| TEXAS INSTRUMENTS INCORPORATED
| Standard Linear and Logic Group
| IBIS Model of SN74AHC138
| 3-LINE TO 8-LINE DECODERS/DEMULTIPLEXERS
| This file contains package information for the following:
|  QFN 16-pin (RGY) package as [Component] AHC138_RGY
|  PDIP 16-pin (N) package as [Component] AHC138_N
|  SOIC 16-pin (D) package as [Component] AHC138_D
|  SOP 16-pin (NS) package as [Component] AHC138_NS
|  SSOP 16-pin (DB) package as [Component] AHC138_DB
|  TSSOP 16-pin (PW) package as [Component] AHC138_PW
|  TVSOP 16-pin (DGV) package as [Component] AHC138_DGV
| This device can be powered at the following Vccs:
|  5 volt Vcc
|  3.3 volt Vcc
| This file provides unique models under the [Model Selector] for each Vcc.
| For operation at a specific Vcc, select the appropriate model after each
| [Model Selector] keyword.
[IBIS Ver]   3.2
[Comment char]  |_char
[File Name]   sn74ahc138.ibs
[File Rev]   1.1 | a_die
[Date]   April 5, 2006
[Source]   Data created from TI-SPICE simulations at TI-SLL.
[Notes]   The following is an IBIS list for the SN74AHC138.
   Please contact sllibis@ti.com with questions and
   comments concerning SLL IBIS models.
   - FILE REV HISTORY
   - 1.1 Release IBIS file on 04/10/06
   - C_comp values are taken at a different test condition
   than the data sheet.
   - Power clamp data deleted as there is no power-clamp diode.
[Disclaimer] Property of Texas Instruments Incorporated.  Unauthorized
   reproduction and/or distribution is strictly prohibited.
   This product is protected under copyright law.
   Created  2006, (C) Copyright  2006, Texas Instruments
   Incorporated, All Rights Reserved
   UNLESS THERE IS A SIGNED, WRITTEN AGREEMENT TO THE
   CONTRARY, TEXAS INSTRUMENTS (TI) IS PROVIDING THE IBIS
   MODELS  AND WITHOUT ANY WARRANTY, EXPRESSED OR
   IMPLIED.  TI assumes no liability for:
   1) the accuracy of the IBIS models provided to your
   company;
   2) the proper functioning of these IBIS Models in your
   design or for any resulting applications; or
   3) infringement of patents, copyrights or intellectual
   property rights resulting from your use of these IBIS
   models.
   TI provides IBIS Models as a service to our customers.
   You and your company shall not distribute, sell or give
   these models to anyone else without prior written
   permission from TI.
   TI reserves the right to make changes to our products or
   to discontinue any semiconductor product or service
   without notice, and advises our customers to obtain the
   latest version of relevant information to verify, before
   placing orders, that the information being relied on is
   current.
   Please be aware that your receipt and use of the IBIS
   information provided shall serve as acceptance of these
   terms and conditions.  If you do not accept these terms,
   you should return or destroy the IBIS models and any
   other accompanying information immediately.
| Component SN74AHC138_RGY 16-PIN QFN
[Component]   SN74AHC138_RGY
[Manufacturer]   Texas Instruments, Inc.
[Package]
|   typ   min   max
R_pkg   3.900e-02   3.700e-02   4.200e-02
L_pkg   8.860e-10   8.430e-10   9.330e-10
C_pkg   3.270e-13   3.140e-13   3.360e-13
[Pin]   signal_name   model_name   R_pin   L_pin   C_pin
1   A   AHC138_IN   4.100e-02   9.250e-10   3.140e-13
2   B   AHC138_IN   4.000e-02   9.000e-10   3.260e-13
3   C   AHC138_IN   3.900e-02   8.820e-10   3.330e-13
4   NG2A   AHC138_IN   4.100e-02   9.150e-10   3.300e-13
5   NG2B   AHC138_IN   4.000e-02   9.000e-10   3.300e-13
6   G1   AHC138_IN   4.000e-02   8.910e-10   3.290e-13
7   Y7   AHC138_OUT   4.100e-02   9.240e-10   3.300e-13
8   GND   GND   4.200e-02   9.330e-10   3.360e-13
9   Y6   AHC138_OUT   3.900e-02   8.850e-10   3.250e-13
10   Y5   AHC138_OUT   3.700e-02   8.430e-10   3.210e-13
11   Y4   AHC138_OUT   3.900e-02   8.730e-10   3.310e-13
12   Y3   AHC138_OUT   3.800e-02   8.550e-10   3.250e-13
13   Y2   AHC138_OUT   3.800e-02   8.530e-10   3.260e-13
14   Y1   AHC138_OUT   3.800e-02   8.570e-10   3.270e-13
15   Y0   AHC138_OUT   3.800e-02   8.540e-10   3.250e-13
16   VCC   POWER   3.900e-02   8.850e-10   3.190e-13
| Component SN74AHC138_N 16-PIN PDIP
[Component]   SN74AHC138_N
[Manufacturer]   Texas Instruments, Inc.
[Package]
|   typ   min   max
R_pkg   5.600e-02   5.200e-02   6.300e-02
L_pkg   7.637e-09   5.451e-09   1.053e-08
C_pkg   5.280e-13   3.350e-13   8.930e-13
[Pin]   signal_name   model_name   R_pin   L_pin   C_pin
1   A   AHC138_IN   5.800e-02   1.053e-08   8.920e-13
2   B   AHC138_IN   6.200e-02   8.759e-09   5.350e-13
3   C   AHC138_IN   5.200e-02   7.146e-09   3.870e-13
4   NG2A   AHC138_IN   5.300e-02   5.451e-09   4.080e-13
5   NG2B   AHC138_IN   5.300e-02   5.513e-09   3.700e-13
6   G1   AHC138_IN   5.300e-02   6.304e-09   3.360e-13
7   Y7   AHC138_OUT   5.700e-02   7.830e-09   5.030e-13
8   GND   GND   5.600e-02   9.581e-09   8.050e-13
9   Y6   AHC138_OUT   5.800e-02   9.603e-09   8.070e-13
10   Y5   AHC138_OUT   6.200e-02   7.864e-09   5.030e-13
11   Y4   AHC138_OUT   5.200e-02   6.295e-09   3.350e-13
12   Y3   AHC138_OUT   5.300e-02   5.499e-09   3.560e-13
13   Y2   AHC138_OUT   5.300e-02   5.452e-09   4.040e-13
14   Y1   AHC138_OUT   5.300e-02   7.156e-09   3.870e-13
15   Y0   AHC138_OUT   6.300e-02   8.740e-09   5.340e-13
16   VCC   POWER   5.600e-02   1.048e-08   8.930e-13
| Component SN74AHC138_D 16-PIN SOIC
[Component]   SN74AHC138_D
[Manufacturer]   Texas Instruments, Inc.
[Package]
|   typ   min   max
R_pkg   3.900e-02   2.800e-02   4.900e-02
L_pkg   3.453e-09   2.350e-09   4.375e-09
C_pkg   5.210e-13   2.540e-13   7.080e-13
[Pin]   signal_name   model_name   R_pin   L_pin   C_pin
1   A   AHC138_IN   4.200e-02   4.336e-09   7.030e-13
2   B   AHC138_IN   4.900e-02   3.778e-09   6.340e-13
3   C   AHC138_IN   2.800e-02   3.449e-09   5.180e-13
4   NG2A   AHC138_IN   2.900e-02   2.393e-09   2.540e-13
5   NG2B   AHC138_IN   2.800e-02   2.350e-09   2.640e-13
6   G1   AHC138_IN   4.800e-02   3.312e-09   4.830e-13
7   Y7   AHC138_OUT   4.300e-02   3.629e-09   6.040e-13
8   GND   GND   4.400e-02   4.375e-09   7.080e-13
9   Y6   AHC138_OUT   4.200e-02   4.336e-09   7.030e-13
10   Y5   AHC138_OUT   4.900e-02   3.778e-09   6.340e-13
11   Y4   AHC138_OUT   2.800e-02   3.449e-09   5.180e-13
12   Y3   AHC138_OUT   2.900e-02   2.393e-09   2.550e-13
13   Y2   AHC138_OUT   2.800e-02   2.350e-09   2.640e-13
14   Y1   AHC138_OUT   4.800e-02   3.312e-09   4.830e-13
15   Y0   AHC138_OUT   4.300e-02   3.629e-09   6.040e-13
16   VCC   POWER   4.400e-02   4.375e-09   7.080e-13
| Component SN74AHC138_NS 16-PIN SOP
[Component]   SN74AHC138_NS
[Manufacturer]   Texas Instruments, Inc.
[Package]
|   typ   min   max
R_pkg   4.200e-02   3.500e-02   4.900e-02
L_pkg   3.147e-09   2.164e-09   4.219e-09
C_pkg   4.040e-13   2.410e-13   5.620e-13
[Pin]   signal_name   model_name   R_pin   L_pin   C_pin
1   A   AHC138_IN   4.900e-02   4.215e-09   5.620e-13
2   B   AHC138_IN   4.600e-02   3.675e-09   4.800e-13
3   C   AHC138_IN   3.700e-02   2.527e-09   3.320e-13
4   NG2A   AHC138_IN   3.500e-02   2.164e-09   2.410e-13
5   NG2B   AHC138_IN   3.500e-02   2.164e-09   2.410e-13
6   G1   AHC138_IN   3.700e-02   2.527e-09   3.320e-13
7   Y7   AHC138_OUT   4.600e-02   3.675e-09   4.800e-13
8   GND   GND   4.900e-02   4.215e-09   5.620e-13
9   Y6   AHC138_OUT   4.900e-02   4.219e-09   5.620e-13
10   Y5   AHC138_OUT   4.600e-02   3.679e-09   4.800e-13
11   Y4   AHC138_OUT   3.700e-02   2.531e-09   3.330e-13
12   Y3   AHC138_OUT   3.500e-02   2.168e-09   2.410e-13
13   Y2   AHC138_OUT   3.500e-02   2.168e-09   2.410e-13
14   Y1   AHC138_OUT   3.700e-02   2.531e-09   3.330e-13
15   Y0   AHC138_OUT   4.600e-02   3.679e-09   4.800e-13
16   VCC   POWER   4.900e-02   4.219e-09   5.620e-13
| Component SN74AHC138_DB 16-PIN SSOP
[Component]   SN74AHC138_DB
[Manufacturer]   Texas Instruments, Inc.
[Package]
|   typ   min   max
R_pkg   4.800e-02   4.600e-02   5.000e-02
L_pkg   3.536e-09   3.213e-09   3.798e-09
C_pkg   3.760e-13   3.140e-13   4.400e-13
[Pin]   signal_name   model_name   R_pin   L_pin   C_pin
1   A   AHC138_IN   4.800e-02   3.797e-09   3.770e-13
2   B   AHC138_IN   4.600e-02   3.723e-09   4.400e-13
3   C   AHC138_IN   4.800e-02   3.409e-09   3.720e-13
4   NG2A   AHC138_IN   4.900e-02   3.213e-09   3.140e-13
5   NG2B   AHC138_IN   4.900e-02   3.213e-09   3.140e-13
6   G1   AHC138_IN   4.800e-02   3.409e-09   3.720e-13
7   Y7   AHC138_OUT   4.600e-02   3.723e-09   4.400e-13
8   GND   GND   4.800e-02   3.798e-09   3.770e-13
9   Y6   AHC138_OUT   4.800e-02   3.797e-09   3.770e-13
10   Y5   AHC138_OUT   4.600e-02   3.725e-09   4.400e-13
11   Y4   AHC138_OUT   4.800e-02   3.409e-09   3.720e-13
12   Y3   AHC138_OUT   4.900e-02   3.214e-09   3.140e-13
13   Y2   AHC138_OUT   5.000e-02   3.216e-09   3.140e-13
14   Y1   AHC138_OUT   4.800e-02   3.409e-09   3.720e-13
15   Y0   AHC138_OUT   4.700e-02   3.729e-09   4.400e-13
16   VCC   POWER   4.800e-02   3.797e-09   3.770e-13
| Component SN74AHC138_PW 16-PIN TSSOP
[Component]   SN74AHC138_PW
[Manufacturer]   Texas Instruments, Inc.
[Package]
|   typ   min   max
R_pkg   4.500e-02   3.800e-02   5.100e-02
L_pkg   2.593e-09   2.447e-09   3.080e-09
C_pkg   2.810e-13   2.430e-13   3.770e-13
[Pin]   signal_name   model_name   R_pin   L_pin   C_pin
1   A   AHC138_IN   4.000e-02   3.080e-09   3.770e-13
2   B   AHC138_IN   3.800e-02   2.458e-09   2.810e-13
3   C   AHC138_IN   5.100e-02   2.512e-09   2.550e-13
4   NG2A   AHC138_IN   5.100e-02   2.447e-09   2.430e-13
5   NG2B   AHC138_IN   5.100e-02   2.447e-09   2.430e-13
6   G1   AHC138_IN   5.100e-02   2.512e-09   2.550e-13
7   Y7   AHC138_OUT   3.800e-02   2.458e-09   2.810e-13
8   GND   GND   4.000e-02   3.080e-09   3.770e-13
9   Y6   AHC138_OUT   3.900e-02   2.832e-09   3.160e-13
10   Y5   AHC138_OUT   3.800e-02   2.460e-09   2.790e-13
11   Y4   AHC138_OUT   5.100e-02   2.512e-09   2.550e-13
12   Y3   AHC138_OUT   5.100e-02   2.447e-09   2.430e-13
13   Y2   AHC138_OUT   5.100e-02   2.447e-09   2.430e-13
14   Y1   AHC138_OUT   5.100e-02   2.512e-09   2.550e-13
15   Y0   AHC138_OUT   3.800e-02   2.459e-09   2.790e-13
16   VCC   POWER   3.900e-02   2.832e-09   3.160e-13
| Component SN74AHC138_DGV 16-PIN TVSOP
[Component]   SN74AHC138_DGV
[Manufacturer]   Texas Instruments, Inc.
[Package]
|   typ   min   max
R_pkg   3.900e-02   3.300e-02   4.500e-02
L_pkg   2.543e-09   2.320e-09   2.938e-09
C_pkg   3.860e-13   3.340e-13   4.490e-13
[Pin]   signal_name   model_name   R_pin   L_pin   C_pin
1   A   AHC138_IN   3.500e-02   2.907e-09   4.170e-13
2   B   AHC138_IN   4.200e-02   2.558e-09   4.460e-13
3   C   AHC138_IN   3.800e-02   2.341e-09   3.450e-13
4   NG2A   AHC138_IN   3.800e-02   2.320e-09   3.340e-13
5   NG2B   AHC138_IN   3.900e-02   2.322e-09   3.340e-13
6   G1   AHC138_IN   3.800e-02   2.353e-09   3.420e-13
7   Y7   AHC138_OUT   4.000e-02   2.536e-09   4.410e-13
8   GND   GND   3.300e-02   2.897e-09   4.180e-13
9   Y6   AHC138_OUT   3.500e-02   2.927e-09   4.190e-13
10   Y5   AHC138_OUT   4.500e-02   2.632e-09   4.490e-13
11   Y4   AHC138_OUT   3.900e-02   2.368e-09   3.470e-13
12   Y3   AHC138_OUT   3.900e-02   2.330e-09   3.350e-13
13   Y2   AHC138_OUT   3.900e-02   2.320e-09   3.350e-13
14   Y1   AHC138_OUT   3.900e-02   2.361e-09   3.450e-13
15   Y0   AHC138_OUT   4.100e-02   2.573e-09   4.460e-13
16   VCC   POWER   3.500e-02   2.938e-09   4.200e-13
| Model AHC138_IN
[Model Selector]   AHC138_IN
AHC138_IN_50   5 volt Vcc
AHC138_IN_33   3.3 volt Vcc
| Model AHC138_OUT
[Model Selector]   AHC138_OUT
AHC138_OUT_50   5 volt Vcc
AHC138_OUT_33   3.3 volt Vcc
| Models and submodels in the file (4): AHC138_IN_50 (Input), AHC138_IN_33 (Input), AHC138_OUT_50 (Output), AHC138_OUT_33 (Output)
